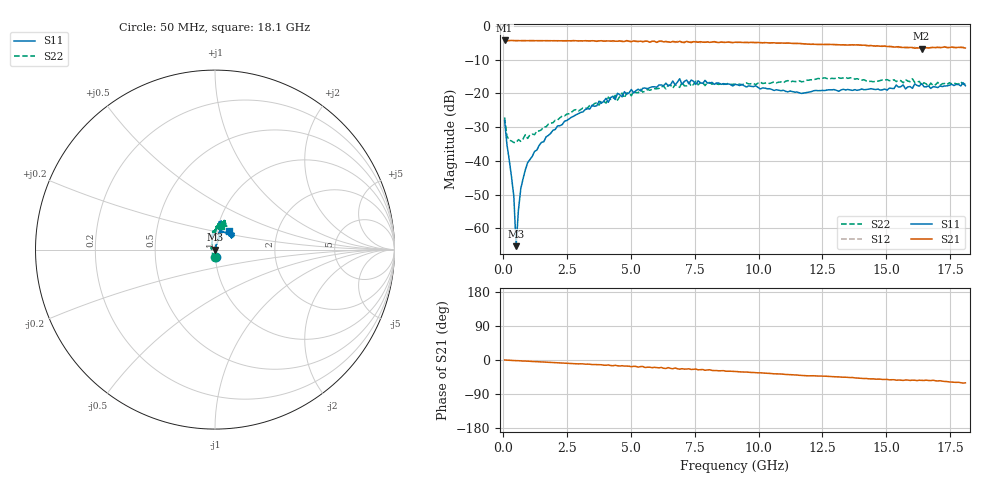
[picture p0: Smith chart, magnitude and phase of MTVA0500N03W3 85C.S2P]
! Network Analyzer HP8720D.06.14 Serial No. US36140669
!  8 Jul 2005  08:27:29
! Frequency  S11  S21  S12  S22
# HZ  S  DB R 50
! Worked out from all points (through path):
!   201 points, 50 MHz to 18.1 GHz, reference 50 ohm
!   highest |S21| = -4.33 dB at 50 MHz (marker M1); lowest = -6.7 dB at 16.39 GHz (marker M2)
!   group delay of S21, straight-line fit = 9.33 ps
!   lowest |S11| = -65.3 dB at 501.2 MHz (marker M3), VSWR 1.00, Z = 50 - j0.0523 ohm
!   |S11| at or under -10 dB: start of sweep to end of sweep
!   |S22| runs from -34.6 to -15.3 dB; largest |S21 - S12| = 0.025
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5e7  -28.03 -83.1  -4.33 0.0  -4.34 -0.0  -27.13 -89.3
1.4025e8  -35.14 -81.9  -4.39 -0.4  -4.37 -0.4  -32.58 -132.2
4.11e8  -50.54 -91.1  -4.37 -1.4  -4.37 -1.4  -34.58 -172.3
5.0125e8  -65.31 -74.7  -4.38 -1.8  -4.37 -1.7  -34.60 175.6
5.915e8  -54.61 100.3  -4.35 -1.8  -4.38 -1.9  -33.72 172.0
6.8175e8  -48.36 93.5  -4.37 -2.3  -4.38 -2.3  -34.25 166.1
9.525e8  -40.55 82.9  -4.38 -3.1  -4.38 -3.1  -33.37 151.1
2.12575e9  -29.64 72.3  -4.39 -7.3  -4.40 -7.2  -27.91 113.3
3.1185e9  -25.51 73.5  -4.44 -10.2  -4.47 -10.6  -24.35 108.2
4.382e9  -21.83 71.9  -4.55 -14.0  -4.51 -15.2  -20.61 98.2
4.47225e9  -19.98 68.7  -4.57 -15.2  -4.47 -14.3  -22.03 101.0
4.65275e9  -21.04 68.8  -4.64 -15.1  -4.47 -16.0  -19.91 99.3
4.743e9  -19.50 72.6  -4.63 -16.1  -4.59 -15.4  -21.35 95.3
6.09675e9  -17.55 73.5  -4.60 -20.7  -4.51 -20.5  -18.54 86.5
6.909e9  -15.68 77.9  -4.55 -24.3  -4.68 -22.9  -18.24 79.5
7.54075e9  -17.35 74.4  -4.78 -23.8  -4.62 -26.1  -16.35 84.3
9.075e9  -17.38 80.2  -4.87 -30.3  -4.84 -30.3  -17.28 76.1
1.21435e10  -19.27 65.1  -5.46 -41.6  -5.41 -41.6  -15.96 74.7
1.512175e10  -18.46 37.7  -6.16 -52.4  -6.00 -52.0  -16.24 73.3
1.602425e10  -18.54 41.2  -6.41 -53.2  -6.57 -55.0  -15.68 68.2
1.638525e10  -17.09 40.7  -6.72 -53.6  -6.55 -53.1  -17.60 69.3
1.81e10  -17.76 51.4  -6.57 -60.4  -6.73 -61.1  -17.27 75.0
